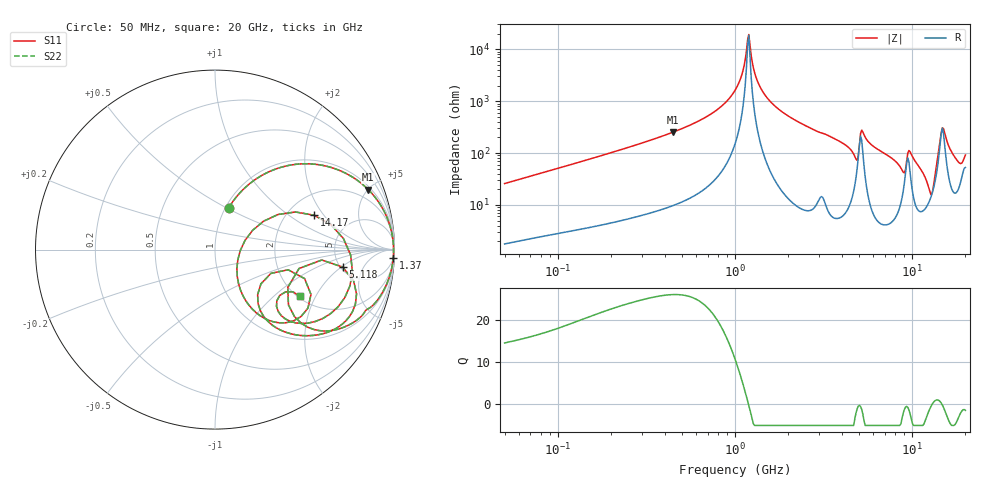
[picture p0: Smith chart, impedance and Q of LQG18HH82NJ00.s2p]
!Murata Part Number: LQG18HH82NJ00
!These Parameters are Measured in Series Mode Connection
!  o--[Z]--o
!Port1  Port2
!  o-------o
!Freq. Start=50[MHz] Stop=20[GHz], 401[Steps]
# Hz S RI R 50
!Freq.(Hz) S11(Real) S11(Imag) S21(Real) S21(Imag) S12(Real) S12(Imag) S22(Real) S22(Imag)
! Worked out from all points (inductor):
!   401 points, 50 MHz to 20 GHz, reference 50 ohm
!   read as one part in series: L = 81.2 nH near 51.52 MHz
!   highest Q = 26 at 445.4 MHz (marker M1), where L = 89.8 nH
!   self-resonance near 1.179 GHz
!   S11 on the Smith chart (normalised r, x): 50 MHz: 1.04, +0.52; 1.37 GHz: 5, -40; 5.118 GHz: 5.23, -2.11; 14.17 GHz: 2.77, +1.61; 20 GHz: 2.05, -1.50
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5e7  0.0766 0.2338  0.9234 -0.2338  0.9234 -0.2338  0.0766 0.2338
1.364002e8  0.3303 0.4461  0.6697 -0.4461  0.6697 -0.4461  0.3303 0.4461
3.721004e8  0.7927 0.3863  0.2073 -0.3863  0.2073 -0.3863  0.7927 0.3863
4.45371e8  0.8542 0.3342  0.1458 -0.3342  0.1458 -0.3342  0.8542 0.3342
7.523192e8  0.9661 0.1591  0.0339 -0.1591  0.0339 -0.1591  0.9661 0.1591
1e9  0.9905 0.0609  0.00947 -0.0609  0.00947 -0.0609  0.9905 0.0609
1.196911e9  0.995 -0.00136  0.00499 0.00136  0.00499 0.00136  0.995 -0.00136
1.369645e9  0.993 -0.0485  0.00703 0.0485  0.00703 0.0485  0.993 -0.0485
1.740566e9  0.977 -0.134  0.023 0.134  0.023 0.134  0.977 -0.134
2.728004e9  0.8874 -0.3024  0.1126 0.3024  0.1126 0.3024  0.8874 -0.3024
4.472136e9  0.5792 -0.4511  0.4208 0.4511  0.4208 0.4511  0.5792 -0.4511
4.81993e9  0.4093 -0.308  0.5907 0.308  0.5907 0.308  0.4093 -0.308
5.117541e9  0.7119 -0.0975  0.2881 0.0975  0.2881 0.0975  0.7119 -0.0975
5.769027e9  0.6914 -0.4285  0.3086 0.4285  0.3086 0.4285  0.6914 -0.4285
7.442007e9  0.4261 -0.4698  0.5739 0.4698  0.5739 0.4698  0.4261 -0.4698
9.178299e9  0.3121 -0.1322  0.6879 0.1322  0.6879 0.1322  0.3121 -0.1322
1.019291e10  0.3968 -0.4075  0.6032 0.4075  0.6032 0.4075  0.3968 -0.4075
1.276073e10  0.1268 -0.0587  0.8732 0.0587  0.8732 0.0587  0.1268 -0.0587
1.417136e10  0.5508 0.1917  0.4492 -0.1917  0.4492 -0.1917  0.5508 0.1917
1.504638e10  0.7656 -0.1197  0.2344 0.1197  0.2344 0.1197  0.7656 -0.1197
1.646126e10  0.5601 -0.4001  0.4399 0.4001  0.4399 0.4001  0.5601 -0.4001
2e10  0.4722 -0.2592  0.5278 0.2592  0.5278 0.2592  0.4722 -0.2592
